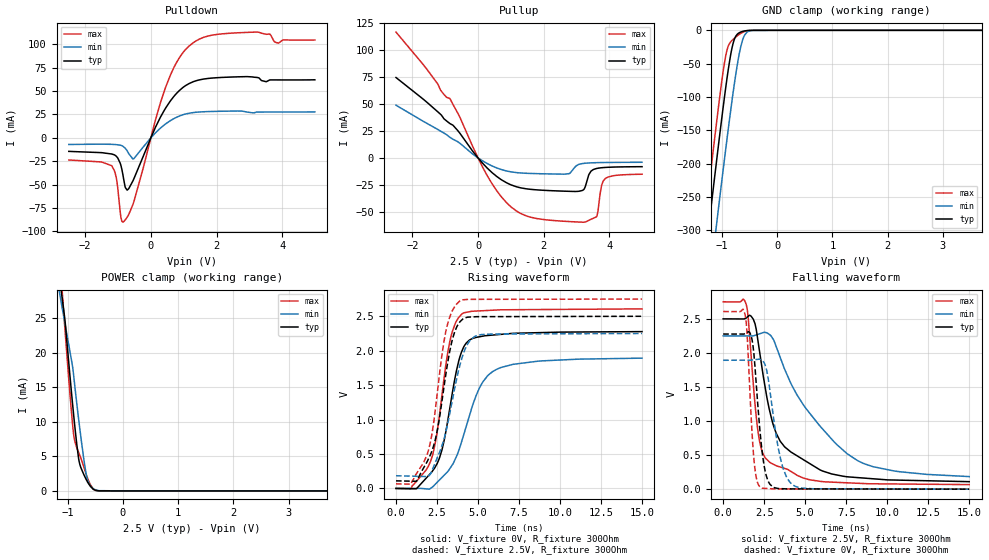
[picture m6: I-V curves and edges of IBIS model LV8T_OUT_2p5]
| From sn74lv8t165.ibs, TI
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[Model]   LV8T_OUT_2p5
Model_type   3-state
Polarity   Non-Inverting
Vmeas = 1.25
Vref = 0
Cref = 15pF
Rref = 1000
|   typ   min   max
C_comp   1.25pF   1.25pF   1.25pF
[Voltage Range]   2.5   2.25   2.75
[Temperature Range]   27   125   -40
[Pullup Reference]   2.5   2.25   2.75
[Pulldown Reference]   0   0   0
[Power Clamp Reference]   2.5   2.25   2.75
[GND Clamp Reference]   0   0   0
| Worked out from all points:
|   slope of the pulldown table from 0 to 0.375 V, typ, clamps not added: 13.7 ohm
|   slope of the pullup table from 0 to 0.375 V, typ, clamps not added: 30.9 ohm
|   GND clamp passes 1 mA (typ) near -0.60 V on its own axis
|   POWER clamp passes 1 mA (typ) near -0.62 V on its own axis
|   falling waveform, V_fixture 2.5V, R_fixture 300Ohm: 20-80 % time 1.7ns typ, 3.57ns min, 687ps max; typ from 2.5 V to 0.11 V
|   rising waveform, V_fixture 0V, R_fixture 300Ohm: 20-80 % time 1.13ns typ, 1.69ns min, 975ps max; typ from 0 V to 2.28 V
|   rising waveform, V_fixture 2.5V, R_fixture 300Ohm: 20-80 % time 1.05ns typ, 1.19ns min, 955ps max; typ from 0.11 V to 2.5 V
|   falling waveform, V_fixture 0V, R_fixture 300Ohm: 20-80 % time 496ps typ, 753ps min, 345ps max; typ from 2.28 V to 0 V
[Pulldown]
|   Voltage   I(typ)   I(min)   I(max)
-2.5V     -14.53mA   -7.127mA   -23.72mA
-1.198V   -17.31mA   -6.98mA    -29.78mA
-1.062V   -19.49mA   -7.279mA   -41.55mA
-914.5mV  -29.45mA   -8.054mA   -84.58mA
-851.5mV  -39.66mA   -9.067mA   -90.36mA
-778mV    -53.26mA   -11.34mA   -87.71mA
-673mV    -54.35mA   -17.06mA   -82.03mA
-515.5mV  -43.66mA   -22.19mA   -68.02mA
429.5mV   30.68mA    14.37mA    52.14mA
1.165V    58.08mA    26.34mA    98.26mA
2.645V    65.29mA    28.67mA    112.4mA
4.997V    62.12mA    27.75mA    104.7mA
[GND Clamp]
|   Voltage   I(typ)   I(min)   I(max)
-2.5V     -1.223A    -1.308A    -1.175A
-1.313V   -348.7mA   -443.1mA   -291.5mA
-1.23V    -288.7mA   -383.5mA   -231.1mA
-1.135V   -222.2mA   -317.2mA   -164.4mA
-1.062V   -171.5mA   -266.3mA   -114.2mA
-977.5mV  -115.5mA   -209.1mA   -61.53mA
-904mV    -69.7mA    -160.4mA   -28.36mA
-778mV    -14.25mA   -82.1mA    -12.14mA
-631mV    -1.745mA   -15.92mA   -3.28mA
-547mV    -376.1uA   -2.828mA   -696.1uA
-431.5mV  -13.18uA   -139.1uA   -11.29uA
8V        0A         0A         0A
[Pullup]
|   Voltage   I(typ)   I(min)   I(max)
-2.5V     74.53mA    48.87mA    116.6mA
-862mV    31.99mA    19.2mA     55.18mA
419mV     -13.38mA   -7.302mA   -23.51mA
1.248V    -27.34mA   -13.8mA    -50.6mA
2.781V    -30.93mA   -14.49mA   -58.95mA
3.18V     -30.12mA   -5.192mA   -59.52mA
3.275V    -25.91mA   -4.857mA   -59.32mA
3.443V    -12.18mA   -4.533mA   -56.79mA
3.611V    -9.773mA   -4.359mA   -54.48mA
3.758V    -9.088mA   -4.264mA   -26.45mA
3.873V    -8.797mA   -4.209mA   -19.21mA
4.997V    -8.087mA   -4.009mA   -15.08mA
[POWER Clamp]
|   Voltage   I(typ)   I(min)   I(max)
-2.5V     122.9mA    97.03mA    154.9mA
-1.125V   29.5mA     27.68mA    31.82mA
-1.051V   24.97mA    24.35mA    23.75mA
-956.5mV  16.59mA    20.13mA    13.96mA
-904mV    12.13mA    17.67mA    9.183mA
-883mV    10.43mA    16.19mA    7.781mA
-830.5mV  6.563mA    12.45mA    6.182mA
-788.5mV  4.183mA    9.634mA    5.343mA
-662.5mV  1.647mA    2.362mA    2.407mA
-589mV    682.9uA    753.1uA    922.8uA
-494.5mV  92.62uA    157.9uA    70.62uA
8V        0A         0A         0A
[Ramp]
R_load = 300
|   typ   min   max
dV/dt_r   1.36615/1.12492e-09   1.13502/1.68632e-09   1.56443/9.71323e-10
dV/dt_f   1.43383/1.67457e-09   1.23927/3.55904e-09   1.60983/6.86303e-10
[Falling Waveform]
V_fixture = 2.5V
V_fixture_min = 2.25V
V_fixture_max = 2.75V
R_fixture = 300Ohm
C_fixture = 0F
|   Time   V(typ)   V(min)   V(max)
0s        2.5V       2.25V      2.75V
1.395ns   2.51V      2.25V      2.719V
1.53ns    2.538V     2.249V     2.505V
1.843ns   2.492V     2.25V      1.528V
2.147ns   2.137V     2.275V     807.6mV
2.825ns   1.16V      2.27V      397.6mV
3.747ns   621.2mV    1.761V     305mV
5.057ns   408.4mV    1.181V     151.5mV
7.557ns   181.7mV    520.7mV    93.42mV
15ns      110.2mV    184.6mV    66.9mV
[Rising Waveform]
V_fixture = 0V
V_fixture_min = 0V
V_fixture_max = 0V
R_fixture = 300Ohm
C_fixture = 0F
|   Time   V(typ)   V(min)   V(max)
0s        155.4uV    367.8uV    79.05uV
907.2ps   -3.762mV   641.5uV    -4.774mV
2.097ns   216.1mV    -1.457mV   388.3mV
2.491ns   354mV      84.33mV    791.2mV
2.807ns   563.4mV    160.5mV    1.366V
3.276ns   1.157V     286mV      2.126V
4.016ns   1.993V     691.4mV    2.533V
5.14ns    2.205V     1.483V     2.579V
6.247ns   2.234V     1.742V     2.592V
15ns      2.277V     1.892V     2.607V
[Rising Waveform]
V_fixture = 2.5V
V_fixture_min = 2.25V
V_fixture_max = 2.75V
R_fixture = 300Ohm
C_fixture = 0F
|   Time   V(typ)   V(min)   V(max)
0s        110.2mV    184.6mV    66.9mV
907.2ps   105.7mV    178.5mV    61.38mV
1.892ns   386.2mV    172.1mV    488.4mV
2.447ns   760.6mV    405.4mV    1.243V
3.029ns   1.642V     811.8mV    2.271V
3.431ns   2.157V     1.275V     2.579V
3.847ns   2.402V     1.743V     2.714V
4.404ns   2.488V     2.112V     2.746V
5.223ns   2.494V     2.235V     2.746V
15ns      2.5V       2.25V      2.75V
[Falling Waveform]
|Gnd
V_fixture = 0V
V_fixture_min = 0V
V_fixture_max = 0V
R_fixture = 300Ohm
C_fixture = 0F
|   Time   V(typ)   V(min)   V(max)
0s        2.277V     1.892V     2.607V
1.331ns   2.285V     1.893V     2.566V
1.456ns   2.301V     1.894V     2.288V
1.708ns   2.248V     1.894V     1.051V
1.892ns   1.934V     1.9V       394.5mV
2.309ns   694.5mV    1.9V       20.8mV
2.849ns   72.22mV    1.449V     7.245mV
3.542ns   7.692mV    401mV      3.269mV
4.34ns    4.129mV    49.13mV    3.047mV
15ns      155.4uV    367.8uV    79uV
